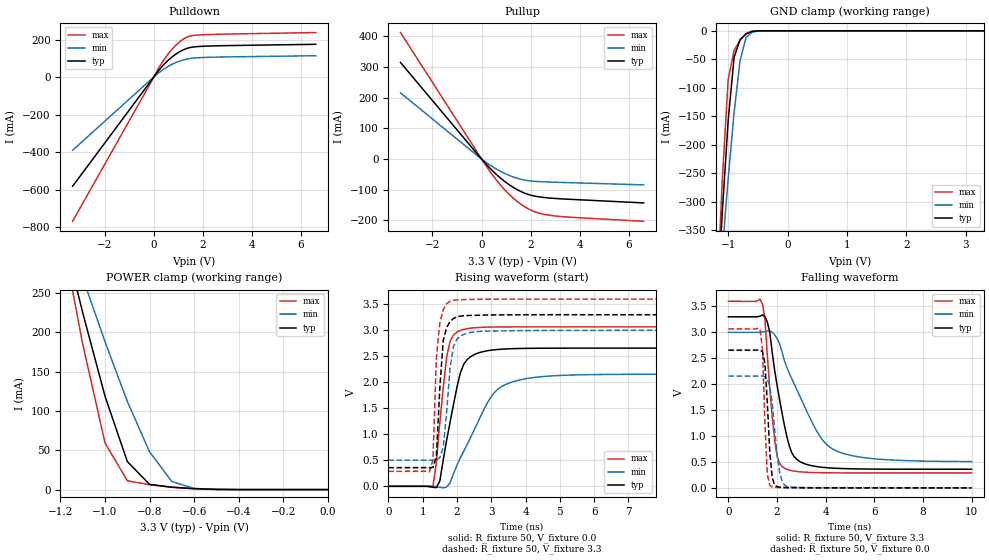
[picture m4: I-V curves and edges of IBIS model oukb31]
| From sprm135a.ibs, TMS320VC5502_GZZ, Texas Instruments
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[Model]   oukb31
Model_type   3-state
Enable   Active-Low
Polarity   Non-Inverting
| signals   A, GZ, Y
Vmeas = 1.5
|   typ   min   max
C_comp   2.5308p   2.4435p   2.7373p
|   typ   min   max
[Temperature Range]   25   -40   125
|   typ   min   max
[Voltage Range]   3.30V   3.00V   3.60V
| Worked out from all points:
|   slope of the pulldown table from 0 to 0.495 V, typ, clamps not added: 6.39 ohm
|   slope of the pullup table from 0 to 0.495 V, typ, clamps not added: 11.7 ohm
|   GND clamp passes 1 mA (typ) near -0.59 V on its own axis
|   POWER clamp passes 1 mA (typ) near -0.58 V on its own axis
|   rising waveform, R_fixture 50, V_fixture 0.0: 20-80 % time 473ps typ, 980ps min, 275ps max; typ from 0 V to 2.66 V
|   falling waveform, R_fixture 50, V_fixture 3.3: 20-80 % time 651ps typ, 1.47ns min, 349ps max; typ from 3.3 V to 0.359 V
|   rising waveform, R_fixture 50, V_fixture 3.3: 20-80 % time 161ps typ, 216ps min, 147ps max; typ from 0.359 V to 3.3 V
|   falling waveform, R_fixture 50, V_fixture 0.0: 20-80 % time 197ps typ, 290ps min, 148ps max; typ from 2.66 V to 0 V
[Pulldown]
|   Voltage   I(typ)   I(min)   I(max)
-3.3V     -581.2mA   -389.7mA   -767.7mA
200mV     34.47mA    21.99mA    47.26mA
600mV     90.59mA    57.59mA    124.9mA
800mV     112.5mA    71.32mA    155.6mA
1.1V      138.1mA    87.04mA    192.2mA
1.4V      154.6mA    97.1mA     215.3mA
1.9V      163.3mA    103.7mA    224.7mA
6.6V      174.6mA    113.7mA    237.1mA
[GND_clamp]
|   Voltage   I(typ)   I(min)   I(max)
-3.3V     -4.769A    -3.596A    -6.191A
-1.2V     -501.9mA   -521.7mA   -498.3mA
-1.1V     -320.2mA   -387.5mA   -263.6mA
-1V       -157mA     -259.3mA   -85.85mA
-900mV    -46.34mA   -142.8mA   -34.26mA
-800mV    -15.6mA    -52.55mA   -16.36mA
-700mV    -5.648mA   -11.79mA   -4.73mA
-600mV    -1.089mA   -2.704mA   -532.9uA
-400mV    -5.549uA   -58.81uA   -554.8nA
3.3V      222pA      3.908uA    133.2pA
[Pullup]
|   Voltage   I(typ)   I(min)   I(max)
-3.3V     314.9mA    215.8mA    412.6mA
-200mV    18.84mA    12.63mA    25.14mA
300mV     -26.49mA   -17.34mA   -35.94mA
600mV     -50.05mA   -32.49mA   -68.19mA
900mV     -70.57mA   -45.36mA   -96.62mA
1.2V      -87.94mA   -55.87mA   -121.1mA
1.5V      -102mA     -63.93mA   -141.6mA
1.8V      -112.8mA   -69.44mA   -157.9mA
2.1V      -120mA     -72.42mA   -170mA
2.7V      -126.8mA   -74.92mA   -182.7mA
3.6V      -131.5mA   -77.25mA   -189.9mA
6.6V      -143.3mA   -84.39mA   -203.3mA
[POWER_clamp]
|   Voltage   I(typ)   I(min)   I(max)
-3.3V     2.98A      2.256A     3.861A
-1.2V     339.4mA    353.6mA    334.4mA
-1.1V     224.8mA    269.3mA    184.9mA
-1V       118.7mA    188mA      59.33mA
-900mV    35.69mA    112.2mA    11.25mA
-800mV    6.565mA    47.93mA    6.232mA
-700mV    2.919mA    10.14mA    3.227mA
-600mV    1.22mA     1.54mA     1.132mA
-400mV    28.23uA    41.58uA    8.826uA
0V        799.4pA    17.85nA    222pA
[Ramp]
|   I(typ)   I(min)   I(max)
dV/dt_r   1.594/0.470n   1.294/0.979n   1.840/0.274n
dV/dt_f   1.764/0.648n   1.496/1.473n   1.987/0.345n
[Rising Waveform]
R_fixture = 50
V_fixture = 0.0
|  pu_on
|  TIME   V(typ)   V(min)   V(max)
0s        1nV        8nV        1nV
1.3ns     -17.77mV   545.8uV    -7.535mV
1.5ns     100.3mV    -19.8mV    1.22V
1.7ns     888.5mV    -12.44mV   2.486V
1.8ns     1.234V     67.1mV     2.79V
2.1ns     2.185V     546.7mV    2.998V
2.4ns     2.494V     941.8mV    3.042V
3ns       2.618V     1.727V     3.063V
3.6ns     2.647V     2.004V     3.066V
9.8ns     2.657V     2.156V     3.067V
[Falling Waveform]
R_fixture = 50
V_fixture = 3.3
V_fixture_min = 3.0
V_fixture_max = 3.6
|  pd_on
|  TIME   V(typ)   V(min)   V(max)
0s        3.3V       3V         3.6V
1.4ns     3.337V     3.006V     3.543V
1.5ns     3.303V     3.015V     3.266V
1.7ns     3.002V     3.028V     1.919V
1.9ns     2.267V     2.953V     925.9mV
2.1ns     1.711V     2.784V     472.9mV
2.3ns     1.212V     2.459V     380.7mV
2.8ns     553.9mV    1.909V     316.7mV
4.3ns     380.8mV    745.5mV    289.9mV
10ns      359.2mV    507.1mV    288mV
[Rising Waveform]
R_fixture = 50
V_fixture = 3.3
V_fixture_min = 3.0
V_fixture_max = 3.6
|  pd_off
|  TIME   V(typ)   V(min)   V(max)
0s        359.2mV    502.7mV    288mV
1.2ns     357.9mV    503.3mV    279.2mV
1.3ns     363.6mV    500mV      508.4mV
1.4ns     574.7mV    502.5mV    2.478V
1.5ns     1.883V     550.4mV    3.138V
1.6ns     2.805V     753.7mV    3.396V
1.8ns     3.168V     2.289V     3.563V
2ns       3.26V      2.828V     3.584V
2.5ns     3.288V     2.97V      3.596V
10ns      3.3V       3V         3.6V
[Falling Waveform]
R_fixture = 50
V_fixture = 0.0
|  pu_off
|  TIME   V(typ)   V(min)   V(max)
0s        2.657V     2.156V     3.067V
1.3ns     2.66V      2.16V      3.063V
1.4ns     2.627V     2.158V     2.673V
1.5ns     2.401V     2.14V      1.257V
1.6ns     1.631V     2.091V     249.4mV
1.7ns     690.9mV    1.965V     47.42mV
1.8ns     198.9mV    1.647V     15.52mV
2.1ns     14.11mV    315.5mV    5.427mV
2.4ns     6.284mV    28.65mV    3.339mV
10ns      1.44uV     58.39uV    397nV
